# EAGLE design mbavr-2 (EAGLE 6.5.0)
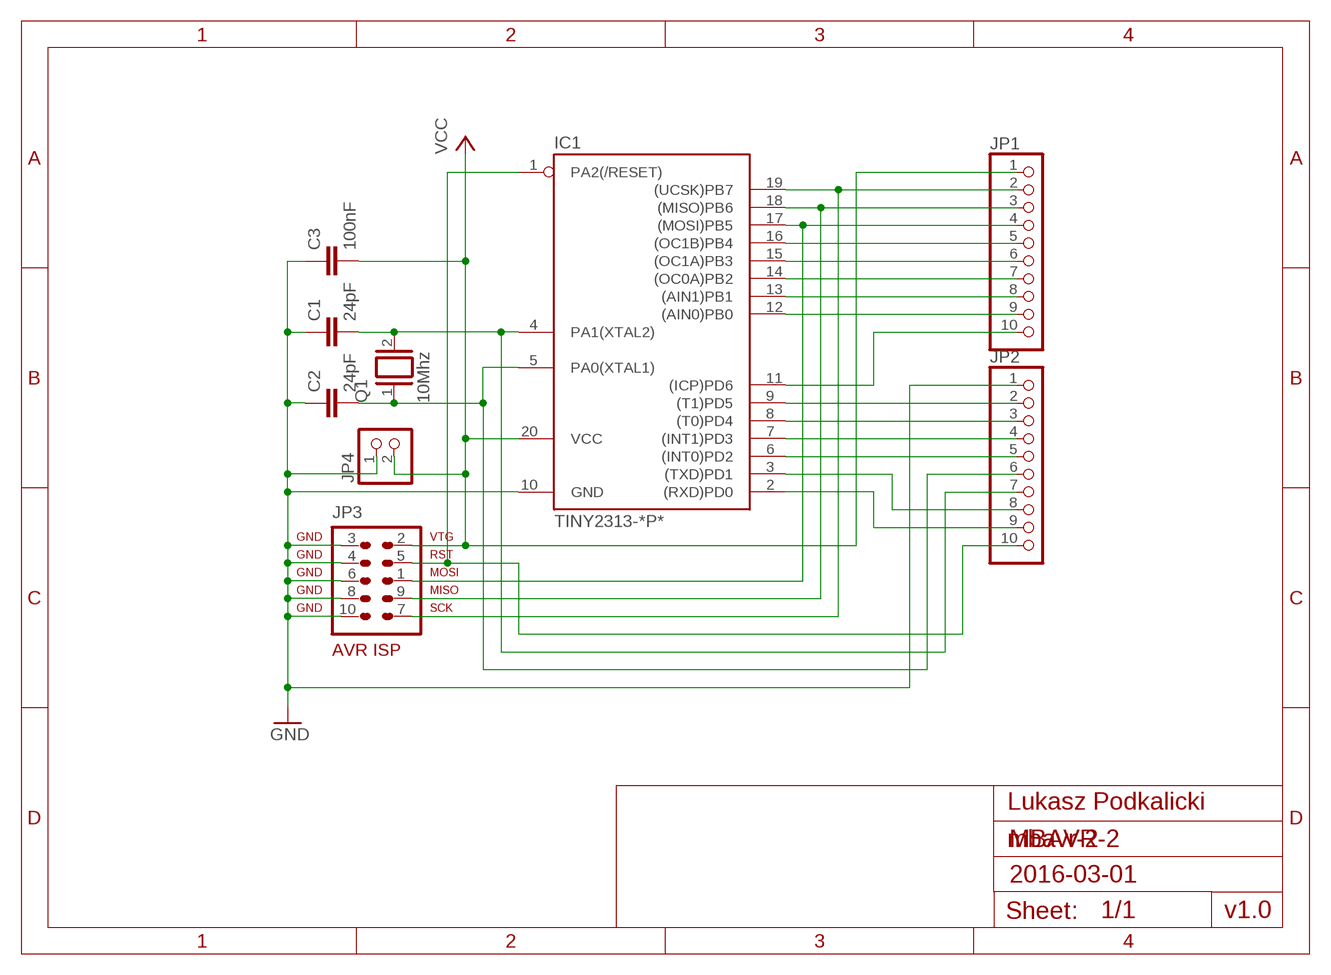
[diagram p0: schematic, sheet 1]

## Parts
C1  24pF  C-EU050-025X075  [C050-025X075]
C2  24pF  C-EU050-025X075  [C050-025X075]
C3  100nF  C-EU050-025X075  [C050-025X075]
IC1  TINY2313-*P*  [DIL20]
JP1  PINHD-1X10  [1X10]
JP2  PINHD-1X10  [1X10]
JP3  AVR-ISP-10  [AVR-ISP-10]
JP4  PINHD-1X2  [1X02]
Q1  10Mhz  XTAL/S  [QS]

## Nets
GND: C1.1 C2.1 C3.1 IC1.10(GND) JP2.1 JP3.3 JP3.4 JP3.6 JP3.8 JP3.10 JP4.1
N$1: C1.2 IC1.4(PA1(XTAL2)) JP2.7 Q1.2
N$2: IC1.11((ICP)PD6) JP1.10
N$5: IC1.2((RXD)PD0) JP2.9
N$6: IC1.3((TXD)PD1) JP2.8
N$7: IC1.6((INT0)PD2) JP2.5
N$8: IC1.7((INT1)PD3) JP2.4
N$9: IC1.8((T0)PD4) JP2.3
N$10: IC1.9((T1)PD5) JP2.2
N$11: IC1.1(PA2(/RESET)) JP2.10 JP3.5
N$12: C2.2 IC1.5(PA0(XTAL1)) JP2.6 Q1.1
N$13: IC1.12((AIN0)PB0) JP1.9
N$14: IC1.13((AIN1)PB1) JP1.8
N$15: IC1.14((OC0A)PB2) JP1.7
N$16: IC1.15((OC1A)PB3) JP1.6
N$17: IC1.16((OC1B)PB4) JP1.5
N$18: IC1.17((MOSI)PB5) JP1.4 JP3.1
N$19: IC1.18((MISO)PB6) JP1.3 JP3.9
N$20: IC1.19((UCSK)PB7) JP1.2 JP3.7
VCC: C3.2 IC1.20(VCC) JP1.1 JP3.2 JP4.2

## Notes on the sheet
- Lukasz Podkalicki
- MBAVR-2
- 2016-03-01
- v1.0

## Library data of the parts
C1-C3 = rcl:C-EU: CAPACITOR, European symbol
IC1 = avr-7:TINY2313*: Atmel Tiny2313 2K Flash, 128 bytes EEPROM, 128 bytes RAM
JP1 JP2 = pinhead:PINHD-1X10: PIN HEADER
JP3 = avr-7:AVR-ISP-10: AVR ISP-10 Serial Programming Header
JP4 = pinhead:PINHD-1X2: PIN HEADER
Q1 = special:XTAL/S: CRYSTAL

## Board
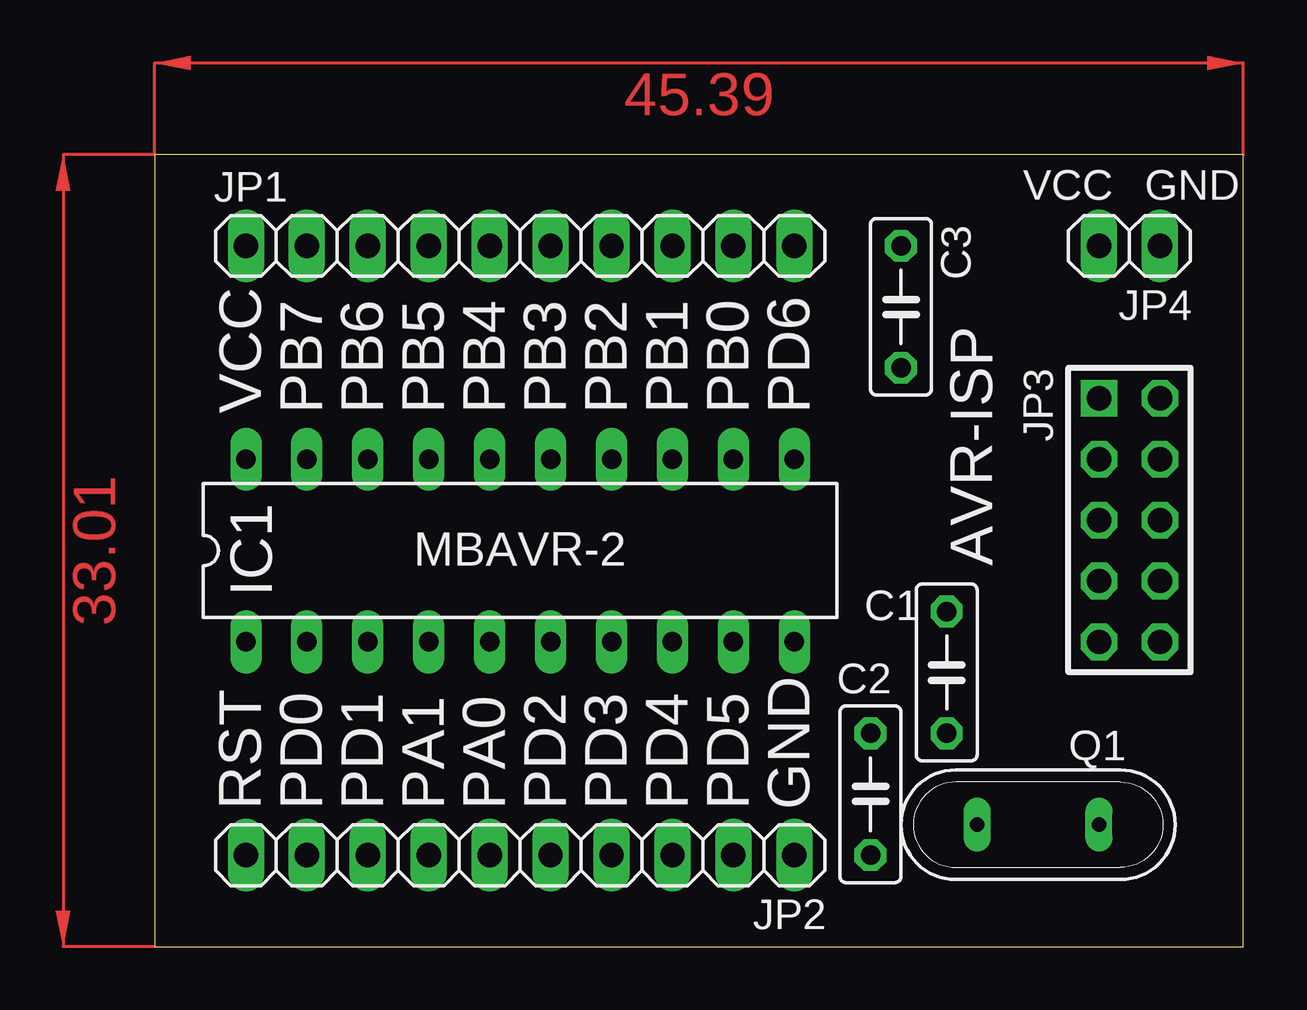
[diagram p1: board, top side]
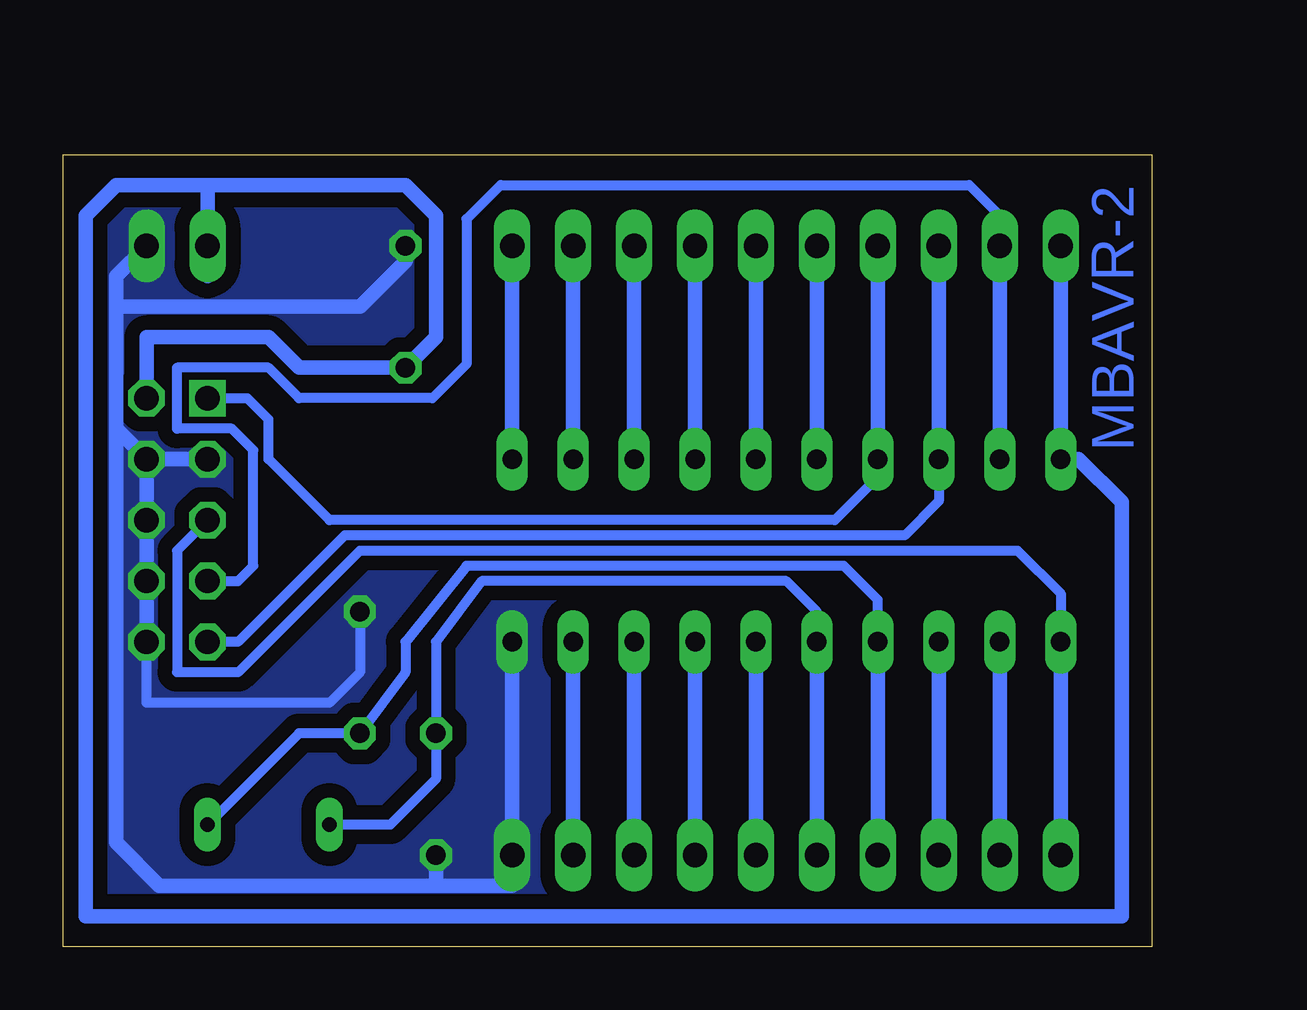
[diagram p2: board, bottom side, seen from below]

Size 45.39 x 33.01 mm. Coordinates in mm from the lower left corner, seen from the top.
Outline: 0,0 45.39,0 45.39,33.01 0,33.01 0,0
Copper layers (1*16): Top 0.035mm / dielectric 1.5mm / Bottom 0.035mm
Design rules "default": minimum track width 10mil, minimum drill 24mil, track to track 8mil, track to pad 8mil, pad to pad 8mil, via to via 8mil, smd to smd 8mil, copper to edge 40mil, drill to drill 8mil, minimum pad ring 10mil, minimum via ring 8mil, stop-mask expansion 4mil, vias tented up to drill 0mil, thermal gap 10mil

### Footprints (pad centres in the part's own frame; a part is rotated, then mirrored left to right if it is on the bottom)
C050-025X075 = drill 0.813 octagon: 1 -2.54,0; 2 2.54,0
DIL20 = drill 0.813 long: 1 -11.43,-3.81; 2 -8.89,-3.81; 3 -6.35,-3.81; 4 -3.81,-3.81; 5 -1.27,-3.81; 6 1.27,-3.81; 7 3.81,-3.81; 8 6.35,-3.81; 9 8.89,-3.81; 10 11.43,-3.81; 11 11.43,3.81; 12 8.89,3.81; 13 6.35,3.81; 14 3.81,3.81; 15 1.27,3.81; 16 -1.27,3.81; 17 -3.81,3.81; 18 -6.35,3.81; 19 -8.89,3.81; 20 -11.43,3.81
1X10 = drill 1.016 long: 1 -11.43,0; 2 -8.89,0; 3 -6.35,0; 4 -3.81,0; 5 -1.27,0; 6 1.27,0; 7 3.81,0; 8 6.35,0; 9 8.89,0; 10 11.43,0
AVR-ISP-10 = drill 1.016 square: 1 -5.08,-1.27 | drill 1.016 octagon: 2 -5.08,1.27; 3 -2.54,-1.27; 4 -2.54,1.27; 5 0,-1.27; 6 0,1.27; 7 2.54,-1.27; 8 2.54,1.27; 9 5.08,-1.27; 10 5.08,1.27
1X02 = drill 1.016 long: 1 -1.27,0; 2 1.27,0
QS = drill 0.61 long: 1 -2.54,0; 2 2.54,0

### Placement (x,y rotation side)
C1  33.02,11.43 270 top
C2  29.84,6.35 90 top
C3  31.11,26.67 270 top
IC1  15.24,16.51 0 top
JP1  15.24,29.21 0 top
JP2  15.24,3.81 180 top
JP3  40.64,17.78 270 top
JP4  40.64,29.21 180 top
Q1  36.83,5.08 0 top

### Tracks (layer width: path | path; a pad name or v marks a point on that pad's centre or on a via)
GND
  Bottom 0.406: C1.1 33.02,11.43 34.29,10.16 41.91,10.16 JP3.10
  Bottom 0.61: JP3.3 JP3.4 | JP3.4 JP3.6 JP3.8 JP3.10 | JP3.4 43.18,21.59 | 43.18,21.59 43.18,26.67 | 43.18,26.67 43.18,27.94 JP4.1 | IC1.10 JP2.1 26.67,2.54 29.84,2.54 | 29.84,2.54 41.38,2.54 43.18,4.34 43.18,21.59 | C2.1 29.84,2.54 | C3.1 31.11,28.57 33.02,26.67 43.18,26.67
  pour Bottom (isolate 0.61, no thermals): -1.27,34.29 -1.27,-1.27 46.99,-1.27 46.99,34.29
N$1
  Bottom 0.406: IC1.4 11.43,14.46 12.85,15.88 28.57,15.88 31.11,12.7 31.11,11.43 C1.2 35.56,8.89 Q1.2
  Bottom 0.61: IC1.4 JP2.7
N$2
  Bottom 0.61: JP1.10 IC1.11
N$5
  Bottom 0.61: IC1.2 JP2.9
N$6
  Bottom 0.61: IC1.3 JP2.8
N$7
  Bottom 0.61: JP2.5 IC1.6
N$8
  Bottom 0.61: JP2.4 IC1.7
N$9
  Bottom 0.61: JP2.3 IC1.8
N$10
  Bottom 0.61: JP2.2 IC1.9
N$11
  Bottom 0.406: JP3.5 40.64,16.51 40.64,11.43 38.1,11.43 33.02,16.51 5.61,16.51 3.81,14.71 IC1.1
  Bottom 0.61: IC1.1 JP2.10
N$12
  Bottom 0.406: IC1.5 13.97,13.97 15.24,15.24 27.94,15.24 29.84,12.7 C2.2 29.84,6.99 31.75,5.08 Q1.1
  Bottom 0.61: IC1.5 JP2.6
N$13
  Bottom 0.61: JP1.9 IC1.12
N$14
  Bottom 0.61: JP1.8 IC1.13
N$15
  Bottom 0.61: JP1.7 IC1.14
N$16
  Bottom 0.61: JP1.6 IC1.15
N$17
  Bottom 0.61: JP1.5 IC1.16
N$18
  Bottom 0.406: JP3.1 37.71,22.86 36.83,21.98 36.83,20.32 34.29,17.78 13.23,17.78 11.43,19.58 IC1.17
  Bottom 0.61: JP1.4 IC1.17
N$19
  Bottom 0.406: IC1.18 8.89,18.57 10.31,17.14 33.65,17.14 38.1,12.7 JP3.9
  Bottom 0.61: JP1.3 IC1.18
N$20
  Bottom 0.406: JP3.7 38.1,15.24 37.46,15.88 37.46,20.69 38.36,21.59 40.64,21.59 40.64,24.13 36.83,24.13 35.56,22.86 30,22.86 28.57,24.28 28.57,30.33 27.16,31.75 7.62,31.75 6.35,30.48 JP1.2
  Bottom 0.61: JP1.2 IC1.19
VCC
  Bottom 0.61: 39.37,27.94 JP4.2 | JP1.1 IC1.20 3.07,20.32 1.27,18.52 1.27,1.27 44.45,1.27 44.45,30.48 43.18,31.75 39.37,31.75 | JP3.2 41.91,25.4 36.83,25.4 35.56,24.13 C3.2 29.84,25.4 29.84,30.48 31.11,31.75 39.37,31.75 | JP4.2 39.37,30.48 | JP4.2 39.37,31.75
(copper drawn outside any net)
  shapes: Top area x2

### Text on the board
Bottom: MBAVR-2
tNames: VCC | GND | VCC | PB7 | PB6 | PB5 | PB4 | PB3 | PB2 | PB1 | PB0 | PD6 | MBAVR-2 | AVR-ISP | RST | PD0 | PD1 | PA1 | PA0 | PD2 | PD3 | PD4 | PD5 | GND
